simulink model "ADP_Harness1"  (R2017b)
settings: Solver=FixedStepDiscrete  StartTime=0.0  StopTime=2  FixedStep=0.01  RelTol=1e-3  EnableMultiTasking=on
undefined symbols (not defined in the file): sigbuilder_block
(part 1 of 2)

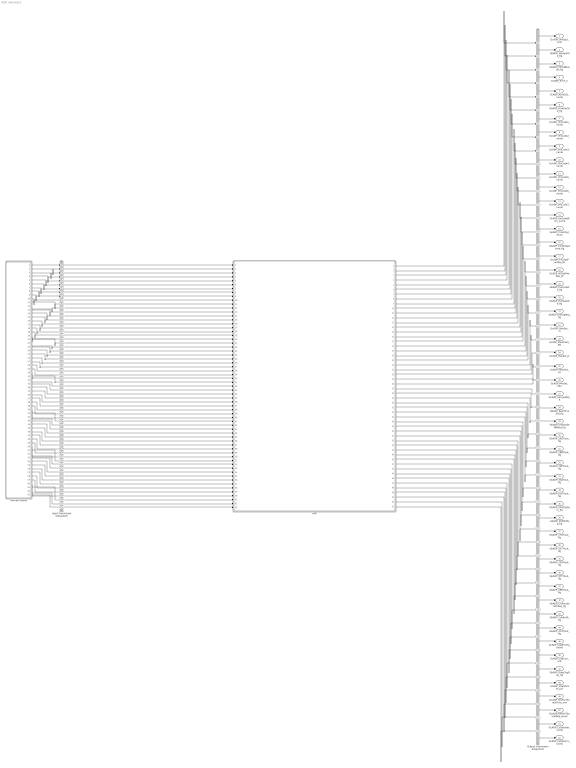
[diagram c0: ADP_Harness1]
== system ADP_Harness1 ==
  ADP : ModelReference  ModelNameDialog=ADP  SimulationMode=Normal  ModelReferenceVersion='M110C112'
  Harness Inputs : Subsystem  Tag=STV Subsys  LoadFcn=sigbuilder_block('load');  StartFcn=sigbuilder_block('start');  StopFcn=sigbuilder_block('stop');  ClipboardFcn=sigbuilder_block('clipboard');  mask(Sigbuilder block){tuvar=[0:10]}
      mask init:
      | if ~strcmp(get_param(bdroot(gcb),'SimulationStatus'),'stopped'),tuvar = sigbuilder_block('maskInit'); end
  Input Conversion Subsystem : Subsystem  Tag=__SLT_ICS__  Description=Signal spec. and routing
  Output Conversion Subsystem : Subsystem  Tag=__SLT_OCS__  Description=Signal spec. and routing
  GcADP_VehSpd_kmh : Outport  OutDataTypeStr=single  PortDimensions=[1]
  GbADP_VehSpdVld_flg : Outport  Port=2  OutDataTypeStr=boolean  PortDimensions=[1]
  GbADP_PtCANBusoff_flg : Outport  Port=3  OutDataTypeStr=boolean  PortDimensions=[1]
  GcADP_EnvT_C : Outport  Port=4  OutDataTypeStr=single  PortDimensions=[1]
  GcADP_AcmDist_numb : Outport  Port=5  OutDataTypeStr=single  PortDimensions=[1]
  GbADP_AcmDistVld_flg : Outport  Port=6  OutDataTypeStr=boolean  PortDimensions=[1]
  GcADP_VinCode1_numb : Outport  Port=7  OutDataTypeStr=uint8  PortDimensions=[1]
  GcADP_VinCode2_numb : Outport  Port=8  OutDataTypeStr=uint8  PortDimensions=[1]
  GcADP_VinCode3_numb : Outport  Port=9  OutDataTypeStr=uint8  PortDimensions=[1]
  GcADP_VinCode4_numb : Outport  Port=10  OutDataTypeStr=uint8  PortDimensions=[1]
  GcADP_VinCode5_numb : Outport  Port=11  OutDataTypeStr=uint8  PortDimensions=[1]
  GcADP_VinCode6_numb : Outport  Port=12  OutDataTypeStr=uint8  PortDimensions=[1]
  GcADP_VinCode7_numb : Outport  Port=13  OutDataTypeStr=uint8  PortDimensions=[1]
  GcADP_VinCodeNum_numb : Outport  Port=14  OutDataTypeStr=uint8  PortDimensions=[1]
  GeADP_CrashSgl_enum : Outport  Port=15  OutDataTypeStr=uint8  PortDimensions=[1]
  GbADP_ChrgStopActive_flg : Outport  Port=16  OutDataTypeStr=boolean  PortDimensions=[1]
  GcADP_PTCOptPwrReq_W : Outport  Port=17  OutDataTypeStr=single  PortDimensions=[1]
  GcADP_ACOptPwrReq_W : Outport  Port=18  OutDataTypeStr=single  PortDimensions=[1]
  GbADP_PreCoolWk_flg : Outport  Port=19  OutDataTypeStr=boolean  PortDimensions=[1]
  GbADP_PreHeatWk_flg : Outport  Port=20  OutDataTypeStr=boolean  PortDimensions=[1]
  GbADP_DischgReq_flg : Outport  Port=21  OutDataTypeStr=boolean  PortDimensions=[1]
  GcADP_YearSet_Yr : Outport  Port=22  OutDataTypeStr=uint16  PortDimensions=[1]
  GcADP_MonthSet_Mn : Outport  Port=23  OutDataTypeStr=uint8  PortDimensions=[1]
  GcADP_DaySet_D : Outport  Port=24  OutDataTypeStr=uint8  PortDimensions=[1]
  GcADP_HourSet_Hr : Outport  Port=25  OutDataTypeStr=uint8  PortDimensions=[1]
  GcADP_MinSet_Min : Outport  Port=26  OutDataTypeStr=uint8  PortDimensions=[1]
  GcADP_SecondSet_S : Outport  Port=27  OutDataTypeStr=uint8  PortDimensions=[1]
  GbADP_RealTimeVld_flg : Outport  Port=28  OutDataTypeStr=boolean  PortDimensions=[1]
  GbADP_OTAmodeONReq_flg : Outport  Port=29  OutDataTypeStr=boolean  PortDimensions=[1]
  GbADP_2ADTiout_flg : Outport  Port=30  OutDataTypeStr=boolean  PortDimensions=[1]
  GbADP_2BBTiout_flg : Outport  Port=31  OutDataTypeStr=boolean  PortDimensions=[1]
  GbADP_2DFTiout_flg : Outport  Port=32  OutDataTypeStr=boolean  PortDimensions=[1]
  GbADP_3AATiout_flg : Outport  Port=33  OutDataTypeStr=boolean  PortDimensions=[1]
  GbADP_050Tiout_flg : Outport  Port=34  OutDataTypeStr=boolean  PortDimensions=[1]
  GbADP_050ChkSum_flg : Outport  Port=35  OutDataTypeStr=boolean  PortDimensions=[1]
  GbADP_050RCMsg_flg : Outport  Port=36  OutDataTypeStr=boolean  PortDimensions=[1]
  GbADP_17DTiout_flg : Outport  Port=37  OutDataTypeStr=boolean  PortDimensions=[1]
  GbADP_2F1Tiout_flg : Outport  Port=38  OutDataTypeStr=boolean  PortDimensions=[1]
  GbADP_195Tiout_flg : Outport  Port=39  OutDataTypeStr=boolean  PortDimensions=[1]
  GbADP_37FTiout_flg : Outport  Port=40  OutDataTypeStr=boolean  PortDimensions=[1]
  GbADP_28DTiout_flg : Outport  Port=41  OutDataTypeStr=boolean  PortDimensions=[1]
  GbADP_OTAmodeOFFReq_flg : Outport  Port=42  OutDataTypeStr=boolean  PortDimensions=[1]
  GbADP_CabErrSt_flg : Outport  Port=43  OutDataTypeStr=boolean  PortDimensions=[1]
  GbADP_3C2Tiout_flg : Outport  Port=44  OutDataTypeStr=boolean  PortDimensions=[1]
  GcADP_CabErrInfo_numb : Outport  Port=45  OutDataTypeStr=uint8  PortDimensions=[1]
  GcADP_CabCurr_mA : Outport  Port=46  OutDataTypeStr=single  PortDimensions=[1]
  GbADP_StopChgReq_flg : Outport  Port=47  OutDataTypeStr=boolean  PortDimensions=[1]
  GcADP_ChgSOCset_pct : Outport  Port=48  OutDataTypeStr=uint8  PortDimensions=[1]
  GcADP_RmPreThemalTime_min : Outport  Port=49  OutDataTypeStr=single  PortDimensions=[1]
  GeADP_RmPreThemalReq_enum : Outport  Port=50  OutDataTypeStr=uint8  PortDimensions=[1]
  GcADP_CsDataVer_numb : Outport  Port=51  OutDataTypeStr=uint8  PortDimensions=[1]
  GcADP_CsDataCrc_numb : Outport  Port=52  OutDataTypeStr=uint8  PortDimensions=[1]
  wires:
  Harness Inputs/1(GcISP_VehSpd_kmh) -> Input Conversion Subsystem/1(Inport_1)
  Harness Inputs/2(GbISP_VehSpdVld_flg) -> Input Conversion Subsystem/2(Inport_2)
  Harness Inputs/3(GbISP_2ADTiout_flg) -> Input Conversion Subsystem/3(Inport_3)
  Harness Inputs/4(GbISP_PtCANBusoff_flg) -> Input Conversion Subsystem/4(Inport_4)
  Harness Inputs/5(GcISP_EnvT_C) -> Input Conversion Subsystem/5(Inport_5)
  Harness Inputs/6(GbISP_2BBTiout_flg) -> Input Conversion Subsystem/6(Inport_6)
  Harness Inputs/7(GcISP_AcmDist_numb) -> Input Conversion Subsystem/7(Inport_7)
  Harness Inputs/8(GbISP_AcmDistVld_flg) -> Input Conversion Subsystem/8(Inport_8)
  Harness Inputs/9(GbISP_2DFTiout_flg) -> Input Conversion Subsystem/9(Inport_9)
  Harness Inputs/10(GcISP_VinCode1_numb) -> Input Conversion Subsystem/10(Inport_10)
  Harness Inputs/11(GcISP_VinCode2_numb) -> Input Conversion Subsystem/11(Inport_11)
  Harness Inputs/12(GcISP_VinCode3_numb) -> Input Conversion Subsystem/12(Inport_12)
  Harness Inputs/13(GcISP_VinCode4_numb) -> Input Conversion Subsystem/13(Inport_13)
  Harness Inputs/14(GcISP_VinCode5_numb) -> Input Conversion Subsystem/14(Inport_14)
  Harness Inputs/15(GcISP_VinCode6_numb) -> Input Conversion Subsystem/15(Inport_15)
  Harness Inputs/16(GcISP_VinCode7_numb) -> Input Conversion Subsystem/16(Inport_16)
  Harness Inputs/17(GcISP_VinCodeNum_numb) -> Input Conversion Subsystem/17(Inport_17)
  Harness Inputs/18(GbISP_3AATiout_flg) -> Input Conversion Subsystem/18(Inport_18)
  Harness Inputs/19(GeISP_CrashSgl_enum) -> Input Conversion Subsystem/19(Inport_19)
  Harness Inputs/20(GbISP_050Tiout_flg) -> Input Conversion Subsystem/20(Inport_20)
  Harness Inputs/21(GbISP_ChrgStopActive_flg) -> Input Conversion Subsystem/21(Inport_21)
  Harness Inputs/22(GbISP_17DTiout_flg) -> Input Conversion Subsystem/22(Inport_22)
  Harness Inputs/23(GcISP_PTCOptPwrReq_W) -> Input Conversion Subsystem/23(Inport_23)
  Harness Inputs/24(GcISP_ACOptPwrReq_W) -> Input Conversion Subsystem/24(Inport_24)
  Harness Inputs/25(GbISP_PreCoolWk_flg) -> Input Conversion Subsystem/25(Inport_25)
  Harness Inputs/26(GbISP_PreHeatWk_flg) -> Input Conversion Subsystem/26(Inport_26)
  Harness Inputs/27(GbISP_2F1Tiout_flg) -> Input Conversion Subsystem/27(Inport_27)
  Harness Inputs/28(GeISP_DischgReq_enum) -> Input Conversion Subsystem/28(Inport_28)
  Harness Inputs/29(GbISP_195Tiout_flg) -> Input Conversion Subsystem/29(Inport_29)
  Harness Inputs/30(GcISP_YearSet_Yr) -> Input Conversion Subsystem/30(Inport_30)
  Harness Inputs/31(GcISP_MonthSet_Mn) -> Input Conversion Subsystem/31(Inport_31)
  Harness Inputs/32(GcISP_DaySet_D) -> Input Conversion Subsystem/32(Inport_32)
  Harness Inputs/33(GcISP_HourSet_Hr) -> Input Conversion Subsystem/33(Inport_33)
  Harness Inputs/34(GcISP_MinSet_Min) -> Input Conversion Subsystem/34(Inport_34)
  Harness Inputs/35(GcISP_SecondSet_S) -> Input Conversion Subsystem/35(Inport_35)
  Harness Inputs/36(GbISP_37FTiout_flg) -> Input Conversion Subsystem/36(Inport_36)
  Harness Inputs/37(GbISP_OTAmodeONReq_flg) -> Input Conversion Subsystem/37(Inport_37)
  Harness Inputs/38(GbISP_28DTiout_flg) -> Input Conversion Subsystem/38(Inport_38)
  Harness Inputs/39(GbVDP_DiagPermit_flg) -> Input Conversion Subsystem/39(Inport_39)
  Harness Inputs/40(GbISP_RcMsg050Err_flg) -> Input Conversion Subsystem/40(Inport_40)
  Harness Inputs/41(GbISP_ChkSumMsg050Err_flg) -> Input Conversion Subsystem/41(Inport_41)
  Harness Inputs/42(GbISP_OTAmodeOFFReq_flg) -> Input Conversion Subsystem/42(Inport_42)
  Harness Inputs/43(GeODP_ObcCcSt_enum) -> Input Conversion Subsystem/43(Inport_43)
  Harness Inputs/44(GbWSM_ACWkUpPrs_flg) -> Input Conversion Subsystem/44(Inport_44)
  Harness Inputs/45(GeVDP_VcuFalutLvl_enum) -> Input Conversion Subsystem/45(Inport_45)
  Harness Inputs/46(GbVDP_VcuChrgDisable_flg) -> Input Conversion Subsystem/46(Inport_46)
  Harness Inputs/47(GbISP_CabErrSt_flg) -> Input Conversion Subsystem/47(Inport_47)
  Harness Inputs/48(GbISP_3C2Tiout_flg) -> Input Conversion Subsystem/48(Inport_48)
  Harness Inputs/49(GcISP_CabErrInfo_numb) -> Input Conversion Subsystem/49(Inport_49)
  Harness Inputs/50(GcISP_CabCurr_mA) -> Input Conversion Subsystem/50(Inport_50)
  Harness Inputs/51(GeISP_StopChgReq_enum) -> Input Conversion Subsystem/51(Inport_51)
  Harness Inputs/52(GcISP_ChgSOCset_pct) -> Input Conversion Subsystem/52(Inport_52)
  Harness Inputs/53(GbFTC_OpenContactor_flg) -> Input Conversion Subsystem/53(Inport_53)
  Harness Inputs/54(GbFTC_PowerDown_flg) -> Input Conversion Subsystem/54(Inport_54)
  Harness Inputs/55(GeMSM_BMUState_enum) -> Input Conversion Subsystem/55(Inport_55)
  Harness Inputs/56(GcODP_ObcFaultLvl_numb) -> Input Conversion Subsystem/56(Inport_56)
  Harness Inputs/57(GbWSM_Kl15WkUpPrs_flg) -> Input Conversion Subsystem/57(Inport_57)
  Harness Inputs/58(GcISP_RmPreThemalTime_min) -> Input Conversion Subsystem/58(Inport_58)
  Harness Inputs/59(GeISP_RmPreThemalReq_enum) -> Input Conversion Subsystem/59(Inport_59)
  Harness Inputs/60(GcISP_CsDataVer_numb) -> Input Conversion Subsystem/60(Inport_60)
  Harness Inputs/61(GcISP_CsDataCrc_numb) -> Input Conversion Subsystem/61(Inport_61)
  Harness Inputs/62(GeUDS_PrjSel_enum) -> Input Conversion Subsystem/62(Inport_62)
  Harness Inputs/63(GeLDP_CC2St_enum) -> Input Conversion Subsystem/63(Inport_63)
  Output Conversion Subsystem/1(Outport_1) -> GcADP_VehSpd_kmh/1
  Output Conversion Subsystem/2(Outport_2) -> GbADP_VehSpdVld_flg/1
  Output Conversion Subsystem/3(Outport_3) -> GbADP_PtCANBusoff_flg/1
  Output Conversion Subsystem/4(Outport_4) -> GcADP_EnvT_C/1
  Output Conversion Subsystem/5(Outport_5) -> GcADP_AcmDist_numb/1
  Output Conversion Subsystem/6(Outport_6) -> GbADP_AcmDistVld_flg/1
  Output Conversion Subsystem/7(Outport_7) -> GcADP_VinCode1_numb/1
  Output Conversion Subsystem/8(Outport_8) -> GcADP_VinCode2_numb/1
  Output Conversion Subsystem/9(Outport_9) -> GcADP_VinCode3_numb/1
  Output Conversion Subsystem/10(Outport_10) -> GcADP_VinCode4_numb/1
  Output Conversion Subsystem/11(Outport_11) -> GcADP_VinCode5_numb/1
  Output Conversion Subsystem/12(Outport_12) -> GcADP_VinCode6_numb/1
  Output Conversion Subsystem/13(Outport_13) -> GcADP_VinCode7_numb/1
  Output Conversion Subsystem/14(Outport_14) -> GcADP_VinCodeNum_numb/1
  Output Conversion Subsystem/15(Outport_15) -> GeADP_CrashSgl_enum/1
  Output Conversion Subsystem/16(Outport_16) -> GbADP_ChrgStopActive_flg/1
  Output Conversion Subsystem/17(Outport_17) -> GcADP_PTCOptPwrReq_W/1
  Output Conversion Subsystem/18(Outport_18) -> GcADP_ACOptPwrReq_W/1
  Output Conversion Subsystem/19(Outport_19) -> GbADP_PreCoolWk_flg/1
  Output Conversion Subsystem/20(Outport_20) -> GbADP_PreHeatWk_flg/1
  Output Conversion Subsystem/21(Outport_21) -> GbADP_DischgReq_flg/1
  Output Conversion Subsystem/22(Outport_22) -> GcADP_YearSet_Yr/1
  Output Conversion Subsystem/23(Outport_23) -> GcADP_MonthSet_Mn/1
  Output Conversion Subsystem/24(Outport_24) -> GcADP_DaySet_D/1
  Output Conversion Subsystem/25(Outport_25) -> GcADP_HourSet_Hr/1
  Output Conversion Subsystem/26(Outport_26) -> GcADP_MinSet_Min/1
  Output Conversion Subsystem/27(Outport_27) -> GcADP_SecondSet_S/1
  Output Conversion Subsystem/28(Outport_28) -> GbADP_RealTimeVld_flg/1
  Output Conversion Subsystem/29(Outport_29) -> GbADP_OTAmodeONReq_flg/1
  Output Conversion Subsystem/30(Outport_30) -> GbADP_2ADTiout_flg/1
  Output Conversion Subsystem/31(Outport_31) -> GbADP_2BBTiout_flg/1
  Output Conversion Subsystem/32(Outport_32) -> GbADP_2DFTiout_flg/1
  Output Conversion Subsystem/33(Outport_33) -> GbADP_3AATiout_flg/1
  Output Conversion Subsystem/34(Outport_34) -> GbADP_050Tiout_flg/1
  Output Conversion Subsystem/35(Outport_35) -> GbADP_050ChkSum_flg/1
  Output Conversion Subsystem/36(Outport_36) -> GbADP_050RCMsg_flg/1
  Output Conversion Subsystem/37(Outport_37) -> GbADP_17DTiout_flg/1
  Output Conversion Subsystem/38(Outport_38) -> GbADP_2F1Tiout_flg/1
  Output Conversion Subsystem/39(Outport_39) -> GbADP_195Tiout_flg/1
  Output Conversion Subsystem/40(Outport_40) -> GbADP_37FTiout_flg/1
  Output Conversion Subsystem/41(Outport_41) -> GbADP_28DTiout_flg/1
  Output Conversion Subsystem/42(Outport_42) -> GbADP_OTAmodeOFFReq_flg/1
  Output Conversion Subsystem/43(Outport_43) -> GbADP_CabErrSt_flg/1
  Output Conversion Subsystem/44(Outport_44) -> GbADP_3C2Tiout_flg/1
  Output Conversion Subsystem/45(Outport_45) -> GcADP_CabErrInfo_numb/1
  Output Conversion Subsystem/46(Outport_46) -> GcADP_CabCurr_mA/1
  Output Conversion Subsystem/47(Outport_47) -> GbADP_StopChgReq_flg/1
  Output Conversion Subsystem/48(Outport_48) -> GcADP_ChgSOCset_pct/1
  Output Conversion Subsystem/49(Outport_49) -> GcADP_RmPreThemalTime_min/1
  Output Conversion Subsystem/50(Outport_50) -> GeADP_RmPreThemalReq_enum/1
  Output Conversion Subsystem/51(Outport_51) -> GcADP_CsDataVer_numb/1
  Output Conversion Subsystem/52(Outport_52) -> GcADP_CsDataCrc_numb/1
  Input Conversion Subsystem/1(Outport_1) -> ADP/1
  Input Conversion Subsystem/2(Outport_2) -> ADP/2
  Input Conversion Subsystem/3(Outport_3) -> ADP/3
  Input Conversion Subsystem/4(Outport_4) -> ADP/4
  Input Conversion Subsystem/5(Outport_5) -> ADP/5
  Input Conversion Subsystem/6(Outport_6) -> ADP/6
  Input Conversion Subsystem/7(Outport_7) -> ADP/7
  Input Conversion Subsystem/8(Outport_8) -> ADP/8
  Input Conversion Subsystem/9(Outport_9) -> ADP/9
  Input Conversion Subsystem/10(Outport_10) -> ADP/10
  Input Conversion Subsystem/11(Outport_11) -> ADP/11
  Input Conversion Subsystem/12(Outport_12) -> ADP/12
  Input Conversion Subsystem/13(Outport_13) -> ADP/13
  Input Conversion Subsystem/14(Outport_14) -> ADP/14
  Input Conversion Subsystem/15(Outport_15) -> ADP/15
  Input Conversion Subsystem/16(Outport_16) -> ADP/16
  Input Conversion Subsystem/17(Outport_17) -> ADP/17
  Input Conversion Subsystem/18(Outport_18) -> ADP/18
  Input Conversion Subsystem/19(Outport_19) -> ADP/19
  Input Conversion Subsystem/20(Outport_20) -> ADP/20
  Input Conversion Subsystem/21(Outport_21) -> ADP/21
  Input Conversion Subsystem/22(Outport_22) -> ADP/22
  Input Conversion Subsystem/23(Outport_23) -> ADP/23
  Input Conversion Subsystem/24(Outport_24) -> ADP/24
  Input Conversion Subsystem/25(Outport_25) -> ADP/25
  Input Conversion Subsystem/26(Outport_26) -> ADP/26
  Input Conversion Subsystem/27(Outport_27) -> ADP/27
  Input Conversion Subsystem/28(Outport_28) -> ADP/28
  Input Conversion Subsystem/29(Outport_29) -> ADP/29
  Input Conversion Subsystem/30(Outport_30) -> ADP/30
  Input Conversion Subsystem/31(Outport_31) -> ADP/31
  Input Conversion Subsystem/32(Outport_32) -> ADP/32
  Input Conversion Subsystem/33(Outport_33) -> ADP/33
  Input Conversion Subsystem/34(Outport_34) -> ADP/34
  Input Conversion Subsystem/35(Outport_35) -> ADP/35
  Input Conversion Subsystem/36(Outport_36) -> ADP/36
  Input Conversion Subsystem/37(Outport_37) -> ADP/37
  Input Conversion Subsystem/38(Outport_38) -> ADP/38
  Input Conversion Subsystem/39(Outport_39) -> ADP/39
  Input Conversion Subsystem/40(Outport_40) -> ADP/40
  Input Conversion Subsystem/41(Outport_41) -> ADP/41
  Input Conversion Subsystem/42(Outport_42) -> ADP/42
  Input Conversion Subsystem/43(Outport_43) -> ADP/43
  Input Conversion Subsystem/44(Outport_44) -> ADP/44
  Input Conversion Subsystem/45(Outport_45) -> ADP/45
  Input Conversion Subsystem/46(Outport_46) -> ADP/46
  Input Conversion Subsystem/47(Outport_47) -> ADP/47
  Input Conversion Subsystem/48(Outport_48) -> ADP/48
  Input Conversion Subsystem/49(Outport_49) -> ADP/49
  Input Conversion Subsystem/50(Outport_50) -> ADP/50
  Input Conversion Subsystem/51(Outport_51) -> ADP/51
  Input Conversion Subsystem/52(Outport_52) -> ADP/52
  Input Conversion Subsystem/53(Outport_53) -> ADP/53
  Input Conversion Subsystem/54(Outport_54) -> ADP/54
  Input Conversion Subsystem/55(Outport_55) -> ADP/55
  Input Conversion Subsystem/56(Outport_56) -> ADP/56
  Input Conversion Subsystem/57(Outport_57) -> ADP/57
  Input Conversion Subsystem/58(Outport_58) -> ADP/58
  Input Conversion Subsystem/59(Outport_59) -> ADP/59
  Input Conversion Subsystem/60(Outport_60) -> ADP/60
  Input Conversion Subsystem/61(Outport_61) -> ADP/61
  Input Conversion Subsystem/62(Outport_62) -> ADP/62
  Input Conversion Subsystem/63(Outport_63) -> ADP/63
  ADP/1 -> Output Conversion Subsystem/1(Inport_1)
  ADP/2 -> Output Conversion Subsystem/2(Inport_2)
  ADP/3 -> Output Conversion Subsystem/3(Inport_3)
  ADP/4 -> Output Conversion Subsystem/4(Inport_4)
  ADP/5 -> Output Conversion Subsystem/5(Inport_5)
  ADP/6 -> Output Conversion Subsystem/6(Inport_6)
  ADP/7 -> Output Conversion Subsystem/7(Inport_7)
  ADP/8 -> Output Conversion Subsystem/8(Inport_8)
  ADP/9 -> Output Conversion Subsystem/9(Inport_9)
  ADP/10 -> Output Conversion Subsystem/10(Inport_10)
  ADP/11 -> Output Conversion Subsystem/11(Inport_11)
  ADP/12 -> Output Conversion Subsystem/12(Inport_12)
  ADP/13 -> Output Conversion Subsystem/13(Inport_13)
  ADP/14 -> Output Conversion Subsystem/14(Inport_14)
  ADP/15 -> Output Conversion Subsystem/15(Inport_15)
  ADP/16 -> Output Conversion Subsystem/16(Inport_16)
  ADP/17 -> Output Conversion Subsystem/17(Inport_17)
  ADP/18 -> Output Conversion Subsystem/18(Inport_18)
  ADP/19 -> Output Conversion Subsystem/19(Inport_19)
  ADP/20 -> Output Conversion Subsystem/20(Inport_20)
  ADP/21 -> Output Conversion Subsystem/21(Inport_21)
  ADP/22 -> Output Conversion Subsystem/22(Inport_22)
  ADP/23 -> Output Conversion Subsystem/23(Inport_23)
  ADP/24 -> Output Conversion Subsystem/24(Inport_24)
  ADP/25 -> Output Conversion Subsystem/25(Inport_25)
  ADP/26 -> Output Conversion Subsystem/26(Inport_26)
  ADP/27 -> Output Conversion Subsystem/27(Inport_27)
  ADP/28 -> Output Conversion Subsystem/28(Inport_28)
  ADP/29 -> Output Conversion Subsystem/29(Inport_29)
  ADP/30 -> Output Conversion Subsystem/30(Inport_30)
  ADP/31 -> Output Conversion Subsystem/31(Inport_31)
  ADP/32 -> Output Conversion Subsystem/32(Inport_32)
  ADP/33 -> Output Conversion Subsystem/33(Inport_33)
  ADP/34 -> Output Conversion Subsystem/34(Inport_34)
  ADP/35 -> Output Conversion Subsystem/35(Inport_35)
  ADP/36 -> Output Conversion Subsystem/36(Inport_36)
  ADP/37 -> Output Conversion Subsystem/37(Inport_37)
  ADP/38 -> Output Conversion Subsystem/38(Inport_38)
  ADP/39 -> Output Conversion Subsystem/39(Inport_39)
  ADP/40 -> Output Conversion Subsystem/40(Inport_40)
  ADP/41 -> Output Conversion Subsystem/41(Inport_41)
  ADP/42 -> Output Conversion Subsystem/42(Inport_42)
  ADP/43 -> Output Conversion Subsystem/43(Inport_43)
  ADP/44 -> Output Conversion Subsystem/44(Inport_44)
  ADP/45 -> Output Conversion Subsystem/45(Inport_45)
  ADP/46 -> Output Conversion Subsystem/46(Inport_46)
  ADP/47 -> Output Conversion Subsystem/47(Inport_47)
  ADP/48 -> Output Conversion Subsystem/48(Inport_48)
  ADP/49 -> Output Conversion Subsystem/49(Inport_49)
  ADP/50 -> Output Conversion Subsystem/50(Inport_50)
  ADP/51 -> Output Conversion Subsystem/51(Inport_51)
  ADP/52 -> Output Conversion Subsystem/52(Inport_52)

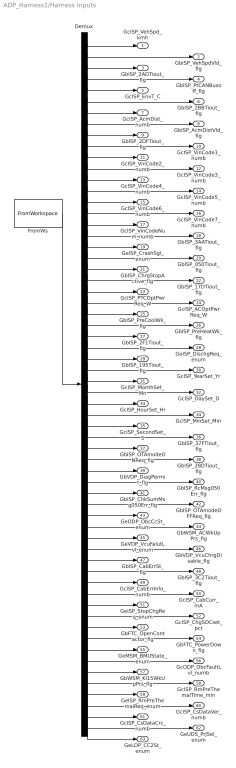
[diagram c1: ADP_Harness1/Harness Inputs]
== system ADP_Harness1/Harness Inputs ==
  Demux : Demux  Tag=STV Demux  Outputs=63
  FromWs : FromWorkspace  Tag=STV FromWs  VariableName=tuvar  SampleTime=0
  GcISP_VehSpd_kmh : Outport  Tag=STV Outport
  GbISP_VehSpdVld_flg : Outport  Tag=STV Outport  Port=2
  GbISP_2ADTiout_flg : Outport  Tag=STV Outport  Port=3
  GbISP_PtCANBusoff_flg : Outport  Tag=STV Outport  Port=4
  GcISP_EnvT_C : Outport  Tag=STV Outport  Port=5
  GbISP_2BBTiout_flg : Outport  Tag=STV Outport  Port=6
  GcISP_AcmDist_numb : Outport  Tag=STV Outport  Port=7
  GbISP_AcmDistVld_flg : Outport  Tag=STV Outport  Port=8
  GbISP_2DFTiout_flg : Outport  Tag=STV Outport  Port=9
  GcISP_VinCode1_numb : Outport  Tag=STV Outport  Port=10
  GcISP_VinCode2_numb : Outport  Tag=STV Outport  Port=11
  GcISP_VinCode3_numb : Outport  Tag=STV Outport  Port=12
  GcISP_VinCode4_numb : Outport  Tag=STV Outport  Port=13
  GcISP_VinCode5_numb : Outport  Tag=STV Outport  Port=14
  GcISP_VinCode6_numb : Outport  Tag=STV Outport  Port=15
  GcISP_VinCode7_numb : Outport  Tag=STV Outport  Port=16
  GcISP_VinCodeNum_numb : Outport  Tag=STV Outport  Port=17
  GbISP_3AATiout_flg : Outport  Tag=STV Outport  Port=18
  GeISP_CrashSgl_enum : Outport  Tag=STV Outport  Port=19
  GbISP_050Tiout_flg : Outport  Tag=STV Outport  Port=20
  GbISP_ChrgStopActive_flg : Outport  Tag=STV Outport  Port=21
  GbISP_17DTiout_flg : Outport  Tag=STV Outport  Port=22
  GcISP_PTCOptPwrReq_W : Outport  Tag=STV Outport  Port=23
  GcISP_ACOptPwrReq_W : Outport  Tag=STV Outport  Port=24
  GbISP_PreCoolWk_flg : Outport  Tag=STV Outport  Port=25
  GbISP_PreHeatWk_flg : Outport  Tag=STV Outport  Port=26
  GbISP_2F1Tiout_flg : Outport  Tag=STV Outport  Port=27
  GeISP_DischgReq_enum : Outport  Tag=STV Outport  Port=28
  GbISP_195Tiout_flg : Outport  Tag=STV Outport  Port=29
  GcISP_YearSet_Yr : Outport  Tag=STV Outport  Port=30
  GcISP_MonthSet_Mn : Outport  Tag=STV Outport  Port=31
  GcISP_DaySet_D : Outport  Tag=STV Outport  Port=32
  GcISP_HourSet_Hr : Outport  Tag=STV Outport  Port=33
  GcISP_MinSet_Min : Outport  Tag=STV Outport  Port=34
  GcISP_SecondSet_S : Outport  Tag=STV Outport  Port=35
  GbISP_37FTiout_flg : Outport  Tag=STV Outport  Port=36
  GbISP_OTAmodeONReq_flg : Outport  Tag=STV Outport  Port=37
  GbISP_28DTiout_flg : Outport  Tag=STV Outport  Port=38
  GbVDP_DiagPermit_flg : Outport  Tag=STV Outport  Port=39
  GbISP_RcMsg050Err_flg : Outport  Tag=STV Outport  Port=40
  GbISP_ChkSumMsg050Err_flg : Outport  Tag=STV Outport  Port=41
  GbISP_OTAmodeOFFReq_flg : Outport  Tag=STV Outport  Port=42
  GeODP_ObcCcSt_enum : Outport  Tag=STV Outport  Port=43
  GbWSM_ACWkUpPrs_flg : Outport  Tag=STV Outport  Port=44
  GeVDP_VcuFalutLvl_enum : Outport  Tag=STV Outport  Port=45
  GbVDP_VcuChrgDisable_flg : Outport  Tag=STV Outport  Port=46
  GbISP_CabErrSt_flg : Outport  Tag=STV Outport  Port=47
  GbISP_3C2Tiout_flg : Outport  Tag=STV Outport  Port=48
  GcISP_CabErrInfo_numb : Outport  Tag=STV Outport  Port=49
  GcISP_CabCurr_mA : Outport  Tag=STV Outport  Port=50
  GeISP_StopChgReq_enum : Outport  Tag=STV Outport  Port=51
  GcISP_ChgSOCset_pct : Outport  Tag=STV Outport  Port=52
  GbFTC_OpenContactor_flg : Outport  Tag=STV Outport  Port=53
  GbFTC_PowerDown_flg : Outport  Tag=STV Outport  Port=54
  GeMSM_BMUState_enum : Outport  Tag=STV Outport  Port=55
  GcODP_ObcFaultLvl_numb : Outport  Tag=STV Outport  Port=56
  GbWSM_Kl15WkUpPrs_flg : Outport  Tag=STV Outport  Port=57
  GcISP_RmPreThemalTime_min : Outport  Tag=STV Outport  Port=58
  GeISP_RmPreThemalReq_enum : Outport  Tag=STV Outport  Port=59
  GcISP_CsDataVer_numb : Outport  Tag=STV Outport  Port=60
  GcISP_CsDataCrc_numb : Outport  Tag=STV Outport  Port=61
  GeUDS_PrjSel_enum : Outport  Tag=STV Outport  Port=62
  GeLDP_CC2St_enum : Outport  Tag=STV Outport  Port=63
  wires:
  FromWs/1 -> Demux/1
  Demux/1 -> GcISP_VehSpd_kmh/1
  Demux/2 -> GbISP_VehSpdVld_flg/1
  Demux/3 -> GbISP_2ADTiout_flg/1
  Demux/4 -> GbISP_PtCANBusoff_flg/1
  Demux/5 -> GcISP_EnvT_C/1
  Demux/6 -> GbISP_2BBTiout_flg/1
  Demux/7 -> GcISP_AcmDist_numb/1
  Demux/8 -> GbISP_AcmDistVld_flg/1
  Demux/9 -> GbISP_2DFTiout_flg/1
  Demux/10 -> GcISP_VinCode1_numb/1
  Demux/11 -> GcISP_VinCode2_numb/1
  Demux/12 -> GcISP_VinCode3_numb/1
  Demux/13 -> GcISP_VinCode4_numb/1
  Demux/14 -> GcISP_VinCode5_numb/1
  Demux/15 -> GcISP_VinCode6_numb/1
  Demux/16 -> GcISP_VinCode7_numb/1
  Demux/17 -> GcISP_VinCodeNum_numb/1
  Demux/18 -> GbISP_3AATiout_flg/1
  Demux/19 -> GeISP_CrashSgl_enum/1
  Demux/20 -> GbISP_050Tiout_flg/1
  Demux/21 -> GbISP_ChrgStopActive_flg/1
  Demux/22 -> GbISP_17DTiout_flg/1
  Demux/23 -> GcISP_PTCOptPwrReq_W/1
  Demux/24 -> GcISP_ACOptPwrReq_W/1
  Demux/25 -> GbISP_PreCoolWk_flg/1
  Demux/26 -> GbISP_PreHeatWk_flg/1
  Demux/27 -> GbISP_2F1Tiout_flg/1
  Demux/28 -> GeISP_DischgReq_enum/1
  Demux/29 -> GbISP_195Tiout_flg/1
  Demux/30 -> GcISP_YearSet_Yr/1
  Demux/31 -> GcISP_MonthSet_Mn/1
  Demux/32 -> GcISP_DaySet_D/1
  Demux/33 -> GcISP_HourSet_Hr/1
  Demux/34 -> GcISP_MinSet_Min/1
  Demux/35 -> GcISP_SecondSet_S/1
  Demux/36 -> GbISP_37FTiout_flg/1
  Demux/37 -> GbISP_OTAmodeONReq_flg/1
  Demux/38 -> GbISP_28DTiout_flg/1
  Demux/39 -> GbVDP_DiagPermit_flg/1
  Demux/40 -> GbISP_RcMsg050Err_flg/1
  Demux/41 -> GbISP_ChkSumMsg050Err_flg/1
  Demux/42 -> GbISP_OTAmodeOFFReq_flg/1
  Demux/43 -> GeODP_ObcCcSt_enum/1
  Demux/44 -> GbWSM_ACWkUpPrs_flg/1
  Demux/45 -> GeVDP_VcuFalutLvl_enum/1
  Demux/46 -> GbVDP_VcuChrgDisable_flg/1
  Demux/47 -> GbISP_CabErrSt_flg/1
  Demux/48 -> GbISP_3C2Tiout_flg/1
  Demux/49 -> GcISP_CabErrInfo_numb/1
  Demux/50 -> GcISP_CabCurr_mA/1
  Demux/51 -> GeISP_StopChgReq_enum/1
  Demux/52 -> GcISP_ChgSOCset_pct/1
  Demux/53 -> GbFTC_OpenContactor_flg/1
  Demux/54 -> GbFTC_PowerDown_flg/1
  Demux/55 -> GeMSM_BMUState_enum/1
  Demux/56 -> GcODP_ObcFaultLvl_numb/1
  Demux/57 -> GbWSM_Kl15WkUpPrs_flg/1
  Demux/58 -> GcISP_RmPreThemalTime_min/1
  Demux/59 -> GeISP_RmPreThemalReq_enum/1
  Demux/60 -> GcISP_CsDataVer_numb/1
  Demux/61 -> GcISP_CsDataCrc_numb/1
  Demux/62 -> GeUDS_PrjSel_enum/1
  Demux/63 -> GeLDP_CC2St_enum/1

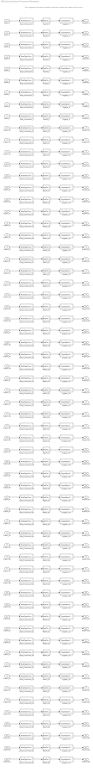
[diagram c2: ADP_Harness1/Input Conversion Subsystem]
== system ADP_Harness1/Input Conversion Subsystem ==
  note: This subsystem has been inserted by Simulink to adapt the output of the source blocks to the interface required by the harnessed component. Modifying the contents of this subsystem may result in compilation and simulation failure.
  Inport_1 : Inport
  Inport_2 : Inport  Port=2
  Inport_3 : Inport  Port=3
  Inport_4 : Inport  Port=4
  Inport_5 : Inport  Port=5
  Inport_6 : Inport  Port=6
  Inport_7 : Inport  Port=7
  Inport_8 : Inport  Port=8
  Inport_9 : Inport  Port=9
  Inport_10 : Inport  Port=10
  Inport_11 : Inport  Port=11
  Inport_12 : Inport  Port=12
  Inport_13 : Inport  Port=13
  Inport_14 : Inport  Port=14
  Inport_15 : Inport  Port=15
  Inport_16 : Inport  Port=16
  Inport_17 : Inport  Port=17
  Inport_18 : Inport  Port=18
  Inport_19 : Inport  Port=19
  Inport_20 : Inport  Port=20
  Inport_21 : Inport  Port=21
  Inport_22 : Inport  Port=22
  Inport_23 : Inport  Port=23
  Inport_24 : Inport  Port=24
  Inport_25 : Inport  Port=25
  Inport_26 : Inport  Port=26
  Inport_27 : Inport  Port=27
  Inport_28 : Inport  Port=28
  Inport_29 : Inport  Port=29
  Inport_30 : Inport  Port=30
  Inport_31 : Inport  Port=31
  Inport_32 : Inport  Port=32
  Inport_33 : Inport  Port=33
  Inport_34 : Inport  Port=34
  Inport_35 : Inport  Port=35
  Inport_36 : Inport  Port=36
  Inport_37 : Inport  Port=37
  Inport_38 : Inport  Port=38
  Inport_39 : Inport  Port=39
  Inport_40 : Inport  Port=40
  Inport_41 : Inport  Port=41
  Inport_42 : Inport  Port=42
  Inport_43 : Inport  Port=43
  Inport_44 : Inport  Port=44
  Inport_45 : Inport  Port=45
  Inport_46 : Inport  Port=46
  Inport_47 : Inport  Port=47
  Inport_48 : Inport  Port=48
  Inport_49 : Inport  Port=49
  Inport_50 : Inport  Port=50
  Inport_51 : Inport  Port=51
  Inport_52 : Inport  Port=52
  Inport_53 : Inport  Port=53
  Inport_54 : Inport  Port=54
  Inport_55 : Inport  Port=55
  Inport_56 : Inport  Port=56
  Inport_57 : Inport  Port=57
  Inport_58 : Inport  Port=58
  Inport_59 : Inport  Port=59
  Inport_60 : Inport  Port=60
  Inport_61 : Inport  Port=61
  Inport_62 : Inport  Port=62
  Inport_63 : Inport  Port=63
  Data_Conversion_1 : DataTypeConversion  OutDataTypeStr=fixdt('ufix16_Sp05625')
  Data_Conversion_{10..17,19,28,31..35,43,45,49,51,55..56,59..63} (26 alike) : DataTypeConversion  OutDataTypeStr=uint8
  Data_Conversion_{2..4,6,8..9,18,20..22,25..27,29,36..42,44,46..48,53..54,57} (28 alike) : DataTypeConversion  OutDataTypeStr=boolean
  Data_Conversion_23 : DataTypeConversion  OutDataTypeStr=uint16
  Data_Conversion_24 : DataTypeConversion  OutDataTypeStr=uint16
  Data_Conversion_30 : DataTypeConversion  OutDataTypeStr=fixdt('ufix8_B2018')
  Data_Conversion_5 : DataTypeConversion  OutDataTypeStr=fixdt('ufix16_En1_Bn80')
  Data_Conversion_50 : DataTypeConversion  OutDataTypeStr=uint32
  Data_Conversion_52 : DataTypeConversion  OutDataTypeStr=fixdt('ufix8_B80')
  Data_Conversion_58 : DataTypeConversion  OutDataTypeStr=fixdt('ufix8_S5')
  Data_Conversion_7 : DataTypeConversion  OutDataTypeStr=fixdt('ufix32_Sp1')
  RateTs_{1..63} (63 alike) : RateTransition  OutPortSampleTime=0.01
  SigSpec_1 : SignalSpecification  OutDataTypeStr=fixdt('ufix16_Sp05625')  Unit=Km/h  Dimensions=[1]  SampleTime=0.01
  SigSpec_{10..17,43,49,56,60..61} (13 alike) : SignalSpecification  OutDataTypeStr=uint8  Unit=numb  Dimensions=[1]  SampleTime=0.01
  SigSpec_{2..4,6,8..9,18,20..22,25..27,29,36..38,40..42,47..48,53..54} (24 alike) : SignalSpecification  OutDataTypeStr=boolean  Unit=flag  Dimensions=[1]  SampleTime=0.01
  SigSpec_{19,28,45,51,55,59,62..63} (8 alike) : SignalSpecification  OutDataTypeStr=uint8  Unit=enum  Dimensions=[1]  SampleTime=0.01
  SigSpec_23 : SignalSpecification  OutDataTypeStr=uint16  Unit=W  Dimensions=[1]  SampleTime=0.01
  SigSpec_24 : SignalSpecification  OutDataTypeStr=uint16  Unit=W  Dimensions=[1]  SampleTime=0.01
  SigSpec_30 : SignalSpecification  OutDataTypeStr=fixdt('ufix8_B2018')  Unit=Yr  Dimensions=[1]  SampleTime=0.01
  SigSpec_31 : SignalSpecification  OutDataTypeStr=uint8  Unit=Min  Dimensions=[1]  SampleTime=0.01
  SigSpec_32 : SignalSpecification  OutDataTypeStr=uint8  Unit=Day  Dimensions=[1]  SampleTime=0.01
  SigSpec_33 : SignalSpecification  OutDataTypeStr=uint8  Unit=Hour  Dimensions=[1]  SampleTime=0.01
  SigSpec_34 : SignalSpecification  OutDataTypeStr=uint8  Unit=Min  Dimensions=[1]  SampleTime=0.01
  SigSpec_35 : SignalSpecification  OutDataTypeStr=uint8  Unit=S  Dimensions=[1]  SampleTime=0.01
  SigSpec_{39,44,46,57} (4 alike) : SignalSpecification  OutDataTypeStr=boolean  Unit=flg  Dimensions=[1]  SampleTime=0.01
  SigSpec_5 : SignalSpecification  OutDataTypeStr=fixdt('ufix16_En1_Bn80')  Unit=℃  Dimensions=[1]  SampleTime=0.01
  SigSpec_50 : SignalSpecification  OutDataTypeStr=uint32  Unit=mA  Dimensions=[1]  SampleTime=0.01
  SigSpec_52 : SignalSpecification  OutDataTypeStr=fixdt('ufix8_B80')  Unit=%  Dimensions=[1]  SampleTime=0.01
  SigSpec_58 : SignalSpecification  OutDataTypeStr=fixdt('ufix8_S5')  Unit=min  Dimensions=[1]  SampleTime=0.01
  SigSpec_7 : SignalSpecification  OutDataTypeStr=fixdt('ufix32_Sp1')  Unit=numb  Dimensions=[1]  SampleTime=0.01
  Outport_1 : Outport
  Outport_2 : Outport  Port=2
  Outport_3 : Outport  Port=3
  Outport_4 : Outport  Port=4
  Outport_5 : Outport  Port=5
  Outport_6 : Outport  Port=6
  Outport_7 : Outport  Port=7
  Outport_8 : Outport  Port=8
  Outport_9 : Outport  Port=9
  Outport_10 : Outport  Port=10
  Outport_11 : Outport  Port=11
  Outport_12 : Outport  Port=12
  Outport_13 : Outport  Port=13
  Outport_14 : Outport  Port=14
  Outport_15 : Outport  Port=15
  Outport_16 : Outport  Port=16
  Outport_17 : Outport  Port=17
  Outport_18 : Outport  Port=18
  Outport_19 : Outport  Port=19
  Outport_20 : Outport  Port=20
  Outport_21 : Outport  Port=21
  Outport_22 : Outport  Port=22
  Outport_23 : Outport  Port=23
  Outport_24 : Outport  Port=24
  Outport_25 : Outport  Port=25
  Outport_26 : Outport  Port=26
  Outport_27 : Outport  Port=27
  Outport_28 : Outport  Port=28
  Outport_29 : Outport  Port=29
  Outport_30 : Outport  Port=30
  Outport_31 : Outport  Port=31
  Outport_32 : Outport  Port=32
  Outport_33 : Outport  Port=33
  Outport_34 : Outport  Port=34
  Outport_35 : Outport  Port=35
  Outport_36 : Outport  Port=36
  Outport_37 : Outport  Port=37
  Outport_38 : Outport  Port=38
  Outport_39 : Outport  Port=39
  Outport_40 : Outport  Port=40
  Outport_41 : Outport  Port=41
  Outport_42 : Outport  Port=42
  Outport_43 : Outport  Port=43
  Outport_44 : Outport  Port=44
  Outport_45 : Outport  Port=45
  Outport_46 : Outport  Port=46
  Outport_47 : Outport  Port=47
  Outport_48 : Outport  Port=48
  Outport_49 : Outport  Port=49
  Outport_50 : Outport  Port=50
  Outport_51 : Outport  Port=51
  Outport_52 : Outport  Port=52
  Outport_53 : Outport  Port=53
  Outport_54 : Outport  Port=54
  Outport_55 : Outport  Port=55
  Outport_56 : Outport  Port=56
  Outport_57 : Outport  Port=57
  Outport_58 : Outport  Port=58
  Outport_59 : Outport  Port=59
  Outport_60 : Outport  Port=60
  Outport_61 : Outport  Port=61
  Outport_62 : Outport  Port=62
  Outport_63 : Outport  Port=63
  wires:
  SigSpec_1/1 -> Outport_1/1
  RateTs_1/1 -> SigSpec_1/1
  Data_Conversion_1/1 -> RateTs_1/1
  Inport_1/1 -> Data_Conversion_1/1
  SigSpec_2/1 -> Outport_2/1
  RateTs_2/1 -> SigSpec_2/1
  Data_Conversion_2/1 -> RateTs_2/1
  Inport_2/1 -> Data_Conversion_2/1
  SigSpec_3/1 -> Outport_3/1
  RateTs_3/1 -> SigSpec_3/1
  Data_Conversion_3/1 -> RateTs_3/1
  Inport_3/1 -> Data_Conversion_3/1
  SigSpec_4/1 -> Outport_4/1
  RateTs_4/1 -> SigSpec_4/1
  Data_Conversion_4/1 -> RateTs_4/1
  Inport_4/1 -> Data_Conversion_4/1
  SigSpec_5/1 -> Outport_5/1
  RateTs_5/1 -> SigSpec_5/1
  Data_Conversion_5/1 -> RateTs_5/1
  Inport_5/1 -> Data_Conversion_5/1
  SigSpec_6/1 -> Outport_6/1
  RateTs_6/1 -> SigSpec_6/1
  Data_Conversion_6/1 -> RateTs_6/1
  Inport_6/1 -> Data_Conversion_6/1
  SigSpec_7/1 -> Outport_7/1
  RateTs_7/1 -> SigSpec_7/1
  Data_Conversion_7/1 -> RateTs_7/1
  Inport_7/1 -> Data_Conversion_7/1
  SigSpec_8/1 -> Outport_8/1
  RateTs_8/1 -> SigSpec_8/1
  Data_Conversion_8/1 -> RateTs_8/1
  Inport_8/1 -> Data_Conversion_8/1
  SigSpec_9/1 -> Outport_9/1
  RateTs_9/1 -> SigSpec_9/1
  Data_Conversion_9/1 -> RateTs_9/1
  Inport_9/1 -> Data_Conversion_9/1
  SigSpec_10/1 -> Outport_10/1
  RateTs_10/1 -> SigSpec_10/1
  Data_Conversion_10/1 -> RateTs_10/1
  Inport_10/1 -> Data_Conversion_10/1
  SigSpec_11/1 -> Outport_11/1
  RateTs_11/1 -> SigSpec_11/1
  Data_Conversion_11/1 -> RateTs_11/1
  Inport_11/1 -> Data_Conversion_11/1
  SigSpec_12/1 -> Outport_12/1
  RateTs_12/1 -> SigSpec_12/1
  Data_Conversion_12/1 -> RateTs_12/1
  Inport_12/1 -> Data_Conversion_12/1
  SigSpec_13/1 -> Outport_13/1
  RateTs_13/1 -> SigSpec_13/1
  Data_Conversion_13/1 -> RateTs_13/1
  Inport_13/1 -> Data_Conversion_13/1
  SigSpec_14/1 -> Outport_14/1
  RateTs_14/1 -> SigSpec_14/1
  Data_Conversion_14/1 -> RateTs_14/1
  Inport_14/1 -> Data_Conversion_14/1
  SigSpec_15/1 -> Outport_15/1
  RateTs_15/1 -> SigSpec_15/1
  Data_Conversion_15/1 -> RateTs_15/1
  Inport_15/1 -> Data_Conversion_15/1
  SigSpec_16/1 -> Outport_16/1
  RateTs_16/1 -> SigSpec_16/1
  Data_Conversion_16/1 -> RateTs_16/1
  Inport_16/1 -> Data_Conversion_16/1
  SigSpec_17/1 -> Outport_17/1
  RateTs_17/1 -> SigSpec_17/1
  Data_Conversion_17/1 -> RateTs_17/1
  Inport_17/1 -> Data_Conversion_17/1
  SigSpec_18/1 -> Outport_18/1
  RateTs_18/1 -> SigSpec_18/1
  Data_Conversion_18/1 -> RateTs_18/1
  Inport_18/1 -> Data_Conversion_18/1
  SigSpec_19/1 -> Outport_19/1
  RateTs_19/1 -> SigSpec_19/1
  Data_Conversion_19/1 -> RateTs_19/1
  Inport_19/1 -> Data_Conversion_19/1
  SigSpec_20/1 -> Outport_20/1
  RateTs_20/1 -> SigSpec_20/1
  Data_Conversion_20/1 -> RateTs_20/1
  Inport_20/1 -> Data_Conversion_20/1
  SigSpec_21/1 -> Outport_21/1
  RateTs_21/1 -> SigSpec_21/1
  Data_Conversion_21/1 -> RateTs_21/1
  Inport_21/1 -> Data_Conversion_21/1
  SigSpec_22/1 -> Outport_22/1
  RateTs_22/1 -> SigSpec_22/1
  Data_Conversion_22/1 -> RateTs_22/1
  Inport_22/1 -> Data_Conversion_22/1
  SigSpec_23/1 -> Outport_23/1
  RateTs_23/1 -> SigSpec_23/1
  Data_Conversion_23/1 -> RateTs_23/1
  Inport_23/1 -> Data_Conversion_23/1
  SigSpec_24/1 -> Outport_24/1
  RateTs_24/1 -> SigSpec_24/1
  Data_Conversion_24/1 -> RateTs_24/1
  Inport_24/1 -> Data_Conversion_24/1
  SigSpec_25/1 -> Outport_25/1
  RateTs_25/1 -> SigSpec_25/1
  Data_Conversion_25/1 -> RateTs_25/1
  Inport_25/1 -> Data_Conversion_25/1
  SigSpec_26/1 -> Outport_26/1
  RateTs_26/1 -> SigSpec_26/1
  Data_Conversion_26/1 -> RateTs_26/1
  Inport_26/1 -> Data_Conversion_26/1
  SigSpec_27/1 -> Outport_27/1
  RateTs_27/1 -> SigSpec_27/1
  Data_Conversion_27/1 -> RateTs_27/1
  Inport_27/1 -> Data_Conversion_27/1
  SigSpec_28/1 -> Outport_28/1
  RateTs_28/1 -> SigSpec_28/1
  Data_Conversion_28/1 -> RateTs_28/1
  Inport_28/1 -> Data_Conversion_28/1
  SigSpec_29/1 -> Outport_29/1
  RateTs_29/1 -> SigSpec_29/1
  Data_Conversion_29/1 -> RateTs_29/1
  Inport_29/1 -> Data_Conversion_29/1
  SigSpec_30/1 -> Outport_30/1
  RateTs_30/1 -> SigSpec_30/1
  Data_Conversion_30/1 -> RateTs_30/1
  Inport_30/1 -> Data_Conversion_30/1
  SigSpec_31/1 -> Outport_31/1
  RateTs_31/1 -> SigSpec_31/1
  Data_Conversion_31/1 -> RateTs_31/1
  Inport_31/1 -> Data_Conversion_31/1
  SigSpec_32/1 -> Outport_32/1
  RateTs_32/1 -> SigSpec_32/1
  Data_Conversion_32/1 -> RateTs_32/1
  Inport_32/1 -> Data_Conversion_32/1
  SigSpec_33/1 -> Outport_33/1
  RateTs_33/1 -> SigSpec_33/1
  Data_Conversion_33/1 -> RateTs_33/1
  Inport_33/1 -> Data_Conversion_33/1
  SigSpec_34/1 -> Outport_34/1
  RateTs_34/1 -> SigSpec_34/1
  Data_Conversion_34/1 -> RateTs_34/1
  Inport_34/1 -> Data_Conversion_34/1
  SigSpec_35/1 -> Outport_35/1
  RateTs_35/1 -> SigSpec_35/1
  Data_Conversion_35/1 -> RateTs_35/1
  Inport_35/1 -> Data_Conversion_35/1
  SigSpec_36/1 -> Outport_36/1
  RateTs_36/1 -> SigSpec_36/1
  Data_Conversion_36/1 -> RateTs_36/1
  Inport_36/1 -> Data_Conversion_36/1
  SigSpec_37/1 -> Outport_37/1
  RateTs_37/1 -> SigSpec_37/1
  Data_Conversion_37/1 -> RateTs_37/1
  Inport_37/1 -> Data_Conversion_37/1
  SigSpec_38/1 -> Outport_38/1
  RateTs_38/1 -> SigSpec_38/1
  Data_Conversion_38/1 -> RateTs_38/1
  Inport_38/1 -> Data_Conversion_38/1
  SigSpec_39/1 -> Outport_39/1
  RateTs_39/1 -> SigSpec_39/1
  Data_Conversion_39/1 -> RateTs_39/1
  Inport_39/1 -> Data_Conversion_39/1
  SigSpec_40/1 -> Outport_40/1
  RateTs_40/1 -> SigSpec_40/1
  Data_Conversion_40/1 -> RateTs_40/1
  Inport_40/1 -> Data_Conversion_40/1
  SigSpec_41/1 -> Outport_41/1
  RateTs_41/1 -> SigSpec_41/1
  Data_Conversion_41/1 -> RateTs_41/1
  Inport_41/1 -> Data_Conversion_41/1
  SigSpec_42/1 -> Outport_42/1
  RateTs_42/1 -> SigSpec_42/1
  Data_Conversion_42/1 -> RateTs_42/1
  Inport_42/1 -> Data_Conversion_42/1
  SigSpec_43/1 -> Outport_43/1
  RateTs_43/1 -> SigSpec_43/1
  Data_Conversion_43/1 -> RateTs_43/1
  Inport_43/1 -> Data_Conversion_43/1
  SigSpec_44/1 -> Outport_44/1
  RateTs_44/1 -> SigSpec_44/1
  Data_Conversion_44/1 -> RateTs_44/1
  Inport_44/1 -> Data_Conversion_44/1
  SigSpec_45/1 -> Outport_45/1
  RateTs_45/1 -> SigSpec_45/1
  Data_Conversion_45/1 -> RateTs_45/1
  Inport_45/1 -> Data_Conversion_45/1
  SigSpec_46/1 -> Outport_46/1
  RateTs_46/1 -> SigSpec_46/1
  Data_Conversion_46/1 -> RateTs_46/1
  Inport_46/1 -> Data_Conversion_46/1
  SigSpec_47/1 -> Outport_47/1
  RateTs_47/1 -> SigSpec_47/1
  Data_Conversion_47/1 -> RateTs_47/1
  Inport_47/1 -> Data_Conversion_47/1
  SigSpec_48/1 -> Outport_48/1
  RateTs_48/1 -> SigSpec_48/1
  Data_Conversion_48/1 -> RateTs_48/1
  Inport_48/1 -> Data_Conversion_48/1
  SigSpec_49/1 -> Outport_49/1
  RateTs_49/1 -> SigSpec_49/1
  Data_Conversion_49/1 -> RateTs_49/1
  Inport_49/1 -> Data_Conversion_49/1
  SigSpec_50/1 -> Outport_50/1
  RateTs_50/1 -> SigSpec_50/1
  Data_Conversion_50/1 -> RateTs_50/1
  Inport_50/1 -> Data_Conversion_50/1
  SigSpec_51/1 -> Outport_51/1
  RateTs_51/1 -> SigSpec_51/1
  Data_Conversion_51/1 -> RateTs_51/1
  Inport_51/1 -> Data_Conversion_51/1
  SigSpec_52/1 -> Outport_52/1
  RateTs_52/1 -> SigSpec_52/1
  Data_Conversion_52/1 -> RateTs_52/1
  Inport_52/1 -> Data_Conversion_52/1
  SigSpec_53/1 -> Outport_53/1
  RateTs_53/1 -> SigSpec_53/1
  Data_Conversion_53/1 -> RateTs_53/1
  Inport_53/1 -> Data_Conversion_53/1
  SigSpec_54/1 -> Outport_54/1
  RateTs_54/1 -> SigSpec_54/1
  Data_Conversion_54/1 -> RateTs_54/1
  Inport_54/1 -> Data_Conversion_54/1
  SigSpec_55/1 -> Outport_55/1
  RateTs_55/1 -> SigSpec_55/1
  Data_Conversion_55/1 -> RateTs_55/1
  Inport_55/1 -> Data_Conversion_55/1
  SigSpec_56/1 -> Outport_56/1
  RateTs_56/1 -> SigSpec_56/1
  Data_Conversion_56/1 -> RateTs_56/1
  Inport_56/1 -> Data_Conversion_56/1
  SigSpec_57/1 -> Outport_57/1
  RateTs_57/1 -> SigSpec_57/1
  Data_Conversion_57/1 -> RateTs_57/1
  Inport_57/1 -> Data_Conversion_57/1
  SigSpec_58/1 -> Outport_58/1
  RateTs_58/1 -> SigSpec_58/1
  Data_Conversion_58/1 -> RateTs_58/1
  Inport_58/1 -> Data_Conversion_58/1
  SigSpec_59/1 -> Outport_59/1
  RateTs_59/1 -> SigSpec_59/1
  Data_Conversion_59/1 -> RateTs_59/1
  Inport_59/1 -> Data_Conversion_59/1
  SigSpec_60/1 -> Outport_60/1
  RateTs_60/1 -> SigSpec_60/1
  Data_Conversion_60/1 -> RateTs_60/1
  Inport_60/1 -> Data_Conversion_60/1
  SigSpec_61/1 -> Outport_61/1
  RateTs_61/1 -> SigSpec_61/1
  Data_Conversion_61/1 -> RateTs_61/1
  Inport_61/1 -> Data_Conversion_61/1
  SigSpec_62/1 -> Outport_62/1
  RateTs_62/1 -> SigSpec_62/1
  Data_Conversion_62/1 -> RateTs_62/1
  Inport_62/1 -> Data_Conversion_62/1
  SigSpec_63/1 -> Outport_63/1
  RateTs_63/1 -> SigSpec_63/1
  Data_Conversion_63/1 -> RateTs_63/1
  Inport_63/1 -> Data_Conversion_63/1
